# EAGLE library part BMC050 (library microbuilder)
BMC050 - Electronic Compass (Three Axis Magnetic Field Sensor and Accelerometer) Support SPI and I2C interfaces Acceleration Range: +/-2g,+/-4g, +/-8g, +/-16g,
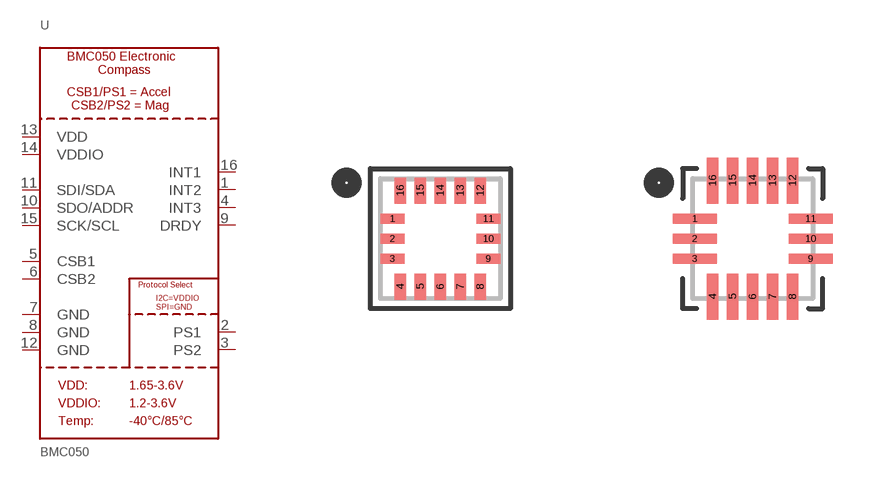
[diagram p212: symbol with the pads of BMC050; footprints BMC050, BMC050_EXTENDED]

Designator prefix U

## BMC050  [BMC050]
1  INT2  out
2  PS1  in
3  PS2  in
4  INT3  out
5  CSB1  in
6  CSB2  in
7  GND  sup
8  GND  sup
9  DRDY  out
10  SDO/ADDR  out
11  SDI/SDA
12  GND  sup
13  VDD  sup
14  VDDIO  sup
15  SCK/SCL  in
16  INT1  out

## BMC050EXT  [BMC050_EXTENDED]
Pads as for BMC050

## Footprint BMC050 (pad centres in mm)
smd 0.6 x 0.25: 1 -1.2,0.5; 2 -1.2,0; 3 -1.2,-0.5; 9 1.2,-0.5; 10 1.2,0; 11 1.2,0.5
smd 0.28 x 0.65: 4 -1,-1.2; 5 -0.5,-1.2; 6 0,-1.2; 7 0.5,-1.2; 8 1,-1.2; 12 1,1.2; 13 0.5,1.2; 14 0,1.2; 15 -0.5,1.2; 16 -1,1.2

## Footprint BMC050_EXTENDED (pad centres in mm)
smd 1.1 x 0.25: 1 -1.45,0.5; 2 -1.45,0; 3 -1.45,-0.5; 9 1.45,-0.5; 10 1.45,0; 11 1.45,0.5
smd 0.28 x 1.15: 4 -1,-1.45; 5 -0.5,-1.45; 6 0,-1.45; 7 0.5,-1.45; 8 1,-1.45; 12 1,1.45; 13 0.5,1.45; 14 0,1.45; 15 -0.5,1.45; 16 -1,1.45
